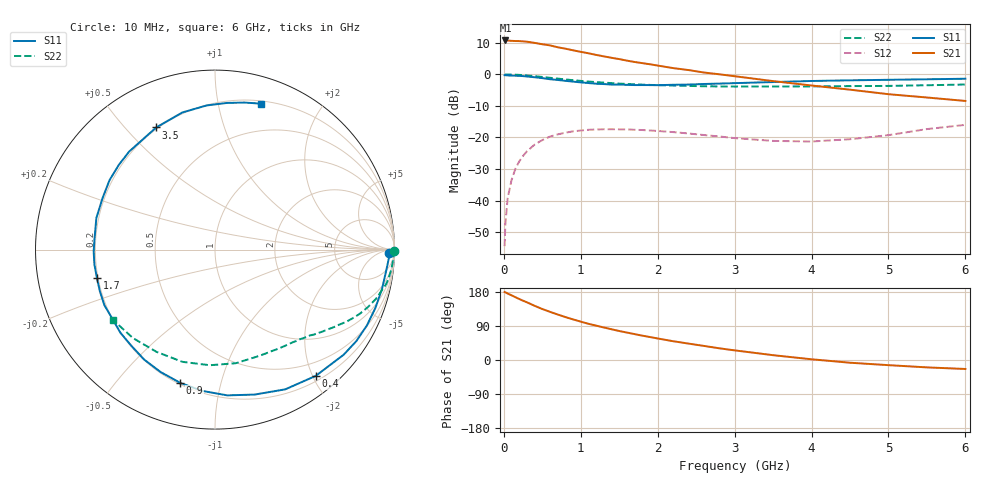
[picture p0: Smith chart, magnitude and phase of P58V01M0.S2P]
! SIEMENS Small Signal Semiconductors
! BFP183
! Si NPN RF Bipolar Junction Transistor in SOT143
! VCE = 8 V  IC = 1 mA
! Common Emitter S-Parameters:  March  1996
# GHz  S  MA  R  50
!  f  S11  S21  S12  S22
! GHz  MAG  ANG  MAG  ANG  MAG  ANG  MAG  ANG
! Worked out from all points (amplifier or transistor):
!   36 points, 10 MHz to 6 GHz, reference 50 ohm
!   highest |S21| = 10.7 dB at 20 MHz (marker M1)
!   |S21| within 3 dB of that: start of sweep to 877 MHz
!   unconditionally stable (mu >= 1): 2.519 GHz to end of sweep
!   at 250 MHz: K = 0.09, MSG = 18.1 dB, |S12| = -25.8 dB
!   at 1.4 GHz: K = 0.53, MSG = 11.3 dB, |S12| = -17.4 dB
!   at 6 GHz: K = 1.06, MAG = 2.3 dB, |S12| = -16.0 dB
!   S11 on the Smith chart (normalised r, x): 10 MHz: 45, -32; 400 MHz: 0.28, -2.05; 900 MHz: 0.21, -0.75; 1.7 GHz: 0.20, -0.11; 3.5 GHz: 0.19, +0.61; 6 GHz: 0.22, +1.34
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0.01  0.971 -1.2  3.437 179.3  0.0019 84.1  0.9999 -0.5
0.02  0.9699 -2.8  3.443 178.7  0.0043 89.0  0.9893 -0.9
0.05  0.9616 -6.7  3.431 175.3  0.011 87.8  0.9949 -2.2
0.1  0.9561 -13.1  3.395 170.7  0.0211 80.5  0.9916 -4.6
0.15  0.9511 -19.9  3.372 165.8  0.0319 78.2  0.9873 -6.9
0.25  0.9382 -32.9  3.326 156.4  0.0511 70.4  0.9729 -11.4
0.3  0.9256 -39.3  3.292 152.3  0.0604 66.2  0.9597 -13.3
0.4  0.9 -51.4  3.152 143.0  0.0772 58.9  0.9374 -17.1
0.5  0.8715 -63.3  3 134.5  0.091 52.1  0.9095 -20.7
0.6  0.8374 -74.7  2.876 127.1  0.1034 45.9  0.8824 -23.9
0.7  0.815 -85.2  2.687 120.0  0.112 40.3  0.8561 -26.6
0.9  0.7672 -104.6  2.404 107.1  0.1252 30.5  0.8079 -31.2
1.1  0.7285 -122.9  2.158 95.5  0.1325 22.5  0.7693 -35.3
1.4  0.6895 -146.1  1.829 81.1  0.1352 12.6  0.7271 -40.6
1.7  0.6766 -166.6  1.571 68.3  0.1325 5.4  0.695 -45.4
1.9  0.676 -179.1  1.444 60.6  0.1292 1.6  0.6808 -48.5
2.2  0.684 165.1  1.257 49.6  0.1218 -2.7  0.6641 -53.5
2.8  0.7141 138.6  1.003 30.9  0.1039 -5.7  0.6436 -64.6
3.5  0.7553 115.7  0.782 12.7  0.0883 0.7  0.6435 -79.6
4.5  0.8045 93.3  0.572 -7.2  0.0939 19.7  0.6512 -106.2
5.5  0.8354 78.7  0.43 -19.5  0.1359 27.5  0.6722 -132.8
6  0.8524 72.6  0.379 -23.7  0.1585 24.9  0.6904 -145.5
